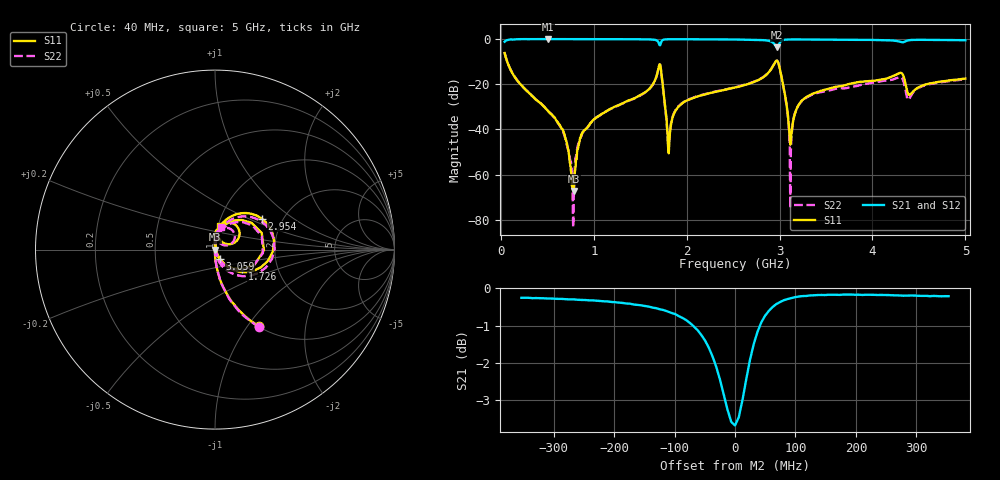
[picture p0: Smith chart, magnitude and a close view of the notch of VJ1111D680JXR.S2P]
! VJ1111D680JXR
! DATE 02/16/2022  11:17
! CAPACITORS MOUNTED IN SERIES ON 25 MIL THICK MICROSTRIP SUBSTRATE
# GHz  S  MA  R  50.00
!  FREQ  S11M  S11A  S21M  S21A  S12M  S12A  S22M  S22A
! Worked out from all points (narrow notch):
!   801 points, 40 MHz to 5 GHz, reference 50 ohm
!   highest |S21| = -0.01 dB at 505 MHz (marker M1); lowest = -3.7 dB at 2.973 GHz (marker M2)
!   notch at M2: 3.5 dB deep, 59.1 MHz wide at half that depth
!   lowest |S11| = -67.3 dB at 784 MHz (marker M3), VSWR 1.00, Z = 50 + j0.0426 ohm
!   |S11| at or under -10 dB: 67.74 MHz to 2.955 GHz (2.888 GHz wide, 191 % of centre); 2.981 GHz to end of sweep
!   |S22| runs from -83.5 to -6.1 dB; largest |S21 - S12| = 0.037
!   S11 on the Smith chart (normalised r, x): 40 MHz: 1.01, -1.13; 1.726 GHz: 1.32, -0.30; 2.954 GHz: 1.57, +0.60; 3.059 GHz: 1.05, -0.10; 5 GHz: 1.02, +0.27
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0.04  0.4905 -60.3  0.8716 29.5  0.872 29.5  0.4978 -60.3
0.505  0.02617 -89.7  0.9984 2.3  1.004 2.3  0.02603 -89.0
0.6786  0.008294 -90.3  0.9974 1.2  1.004 1.0  0.007917 -88.6
0.784  0.0004333 79.3  0.9963 0.9  1.004 0.7  0.0003027 88.4
0.8708  0.007764 89.5  0.9964 0.6  1.003 0.5  0.007613 84.0
1.5776  0.07228 83.5  0.9843 -2.2  0.9915 -2.4  0.07173 79.7
1.6954  0.2212 48.4  0.8524 -8.3  0.8597 -8.5  0.2178 44.7
1.7264  0.1868 -36.1  0.8605 9.9  0.8672 9.8  0.1826 -39.3
1.8132  0.005379 65.7  0.9907 2.0  0.998 1.8  0.006941 58.2
1.962  0.03913 89.9  0.9895 0.2  0.9973 -0.0  0.0395 84.2
2.52  0.08451 84.8  0.9762 -1.9  0.9854 -2.1  0.08528 80.6
2.954  0.3136 33.4  0.7199 -7.7  0.7256 -7.9  0.3138 26.3
2.9726  0.3328 7.9  0.6541 3.0  0.6588 2.8  0.3321 0.4
3.0594  0.05608 -62.4  0.9676 6.6  0.9759 6.4  0.05382 -75.0
3.0966  0.01446 -55.8  0.9785 4.3  0.9871 4.1  0.01305 -81.2
3.1214  0.005425 49.2  0.9798 3.4  0.9891 3.2  0.003409 98.0
3.1896  0.03057 90.4  0.9807 1.9  0.9891 1.6  0.03034 91.8
3.3508  0.06118 89.7  0.9765 0.3  0.9831 0.0  0.0588 86.5
4.1754  0.1383 75.6  0.9406 -3.0  0.9497 -3.3  0.1219 70.7
4.3118  0.177 43.6  0.8537 -1.8  0.8609 -2.1  0.1412 40.9
4.3924  0.05823 45.9  0.9419 2.5  0.9511 2.4  0.04578 60.3
5  0.1335 78.7  0.9426 -3.1  0.9506 -3.4  0.1291 75.6
